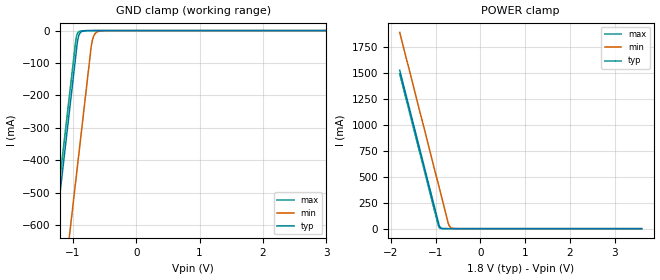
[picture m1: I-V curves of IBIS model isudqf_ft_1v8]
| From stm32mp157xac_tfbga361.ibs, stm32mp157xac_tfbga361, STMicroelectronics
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[Model]   isudqf_ft_1v8
Model_type Input
Polarity   Non-Inverting
Enable   Active-Low
| CAP_THRESHOLD on pad IOFT is "UDTCAPC" :
| Rising=20.00f vddiom   Falling=80.00f vddiom
| C_comp min and max val. don't necessarily correlate with the min and max pvt
| but are the smallest and greatest pad capacitance found.
| var   typ   min   max
C_comp   1.07589pF  1.07188pF  1.08655pF
|C_comp_pullup   479.09500fF  456.27500fF  471.41000fF
|C_comp_pulldown   596.79005fF  615.60000fF  615.13506fF
Vinl = 640.0mV
Vinh = 1.2V
[Model Spec]
| TIME_THRESHOLD on pin ZIV11 is "CMOS" :
| Rising=40.00f vdd   Falling=60.00f vdd
Vinl 864.60000mV 771.60000mV 950.60000mV
Vinh 864.40000mV 771.40000mV 950.40000mV
| variable   typ   min   max
[Temperature Range] 25.0 140.0 -40.0
| variable   typ   min   max
[Voltage Range] 1.8V 1.6V 2.0V
| variable   typ   min   max
[POWER Clamp Reference] 1.8V 1.6V 2.0V
| variable   typ   min   max
[GND Clamp Reference] 0V 0V 0V
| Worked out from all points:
|   GND clamp passes 1 mA (typ) near -0.82 V on its own axis
|   POWER clamp passes 1 mA (typ) near -0.83 V on its own axis
[POWER Clamp]
-1.8V     1.529A     1.894A     1.494A
-940mV    66.83mA    432.1mA    31.5mA
-910mV    22.88mA    381.1mA    7.077mA
-880mV    7.117mA    330.1mA    1.59mA
-720mV    14.05uA    58.12mA    553.9nA
-700mV    6.452uA    33.14mA    204.9nA
-670mV    2.007uA    14.27mA    46.18nA
-610mV    194.5nA    2.645mA    2.401nA
-500mV    2.798nA    120.4uA    39.74pA
3.6V      0A         0A         0A
[GND Clamp]
-1.8V     -1.517A    -1.902A    -1.469A
-1.49V    -990.4mA   -1.375A    -942.4mA
-1.27V    -616.4mA   -1.001A    -568.4mA
-1.2V     -497.4mA   -881.9mA   -449.4mA
-960mV    -89.41mA   -473.9mA   -41.39mA
-930mV    -38.41mA   -422.9mA   -10.17mA
-900mV    -12.55mA   -371.9mA   -2.962mA
-850mV    -2.3mA     -286.9mA   -724.3uA
-710mV    -61.31uA   -49.97mA   -15.96uA
-670mV    -19.6uA    -16.72mA   -8.179uA
-610mV    -6.395uA   -3.464mA   -5.482uA
3.6V      109pA      40.76nA    28.8pA
